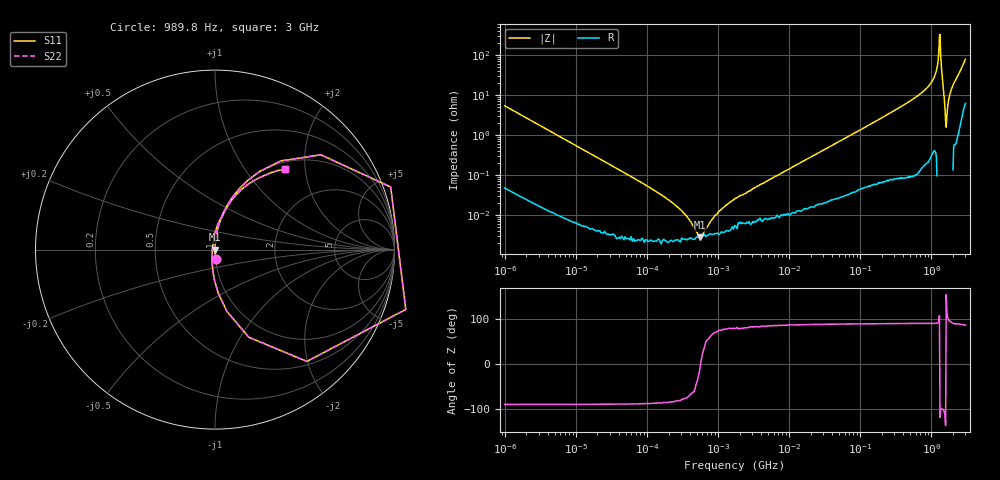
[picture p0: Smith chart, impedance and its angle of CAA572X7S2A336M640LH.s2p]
! S-Parameter Data Generated by TDK Corporation
! Copyright(C) 2020 TDK Corporation.
! All Rights Reserved.
! TDK P/N: CAA572X7S2A336M640LH (Multilayer Ceramic Chip Capacitor)
! Property: C=33uF
! Size(LxWxT): 6x5x6.4mm
! Model Type: s2p (Touchstone File Format Version 1.0)
! Frequency: DC=Yes Start=0.000989846MHz Stop=3000MHz 463points Log-sweep
! Model Generated on Nov. 18, 2020
! Port Assignments:
!  1 ---| |--- 2
! Applicable Conditions:
!  Temperature = 25 degC
!  DC Bias Voltage = 0 V
!  Small Signal Operation
! Terms and conditions regarding TDK Simulation Models
! (1)This simulation model is being provided solely for informational purposes. Please refer to the specifications of the products in terms of detailed characteristics of such products.
! (2)In no event shall TDK Corporation of any of its subsidiaries be liable for any loss or damage arising, directly or indirectly,
!  From any information contained in this simulation model, including, but not limited to loss or damages arising from any inaccuracies, omissions or errors in connection with such information.
! (3)Any and all copyrights on this simulation model are owned by TDK Corporation.
!  Duplication or redistribution of this simulation model without prior written permission from TDK Corporation is prohibited.
! (4)This simulation model is subject to any modification or change without any prior notice.
! (5)Neither TDK Corporation nor any of its subsidiaries shall make any warranty, express or implied,
!  Including but not limited to the correctness, implied warranties of merchantability and fitness for a particular purpose with respect to this simulation models.
! (6)The use of this simulation model shall be deemed to have consented to the terms and conditions hereof.
# Hz S MA R 50
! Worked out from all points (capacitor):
!   462 points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, 989.8 Hz to 3 GHz, reference 50 ohm
!   read as one part in series: C = 29.8 uF near 1.07 kHz
!   lowest |Z| = 2.71 mohm at 550.5 kHz (marker M1)
!   series resonance near 565.4 kHz, so ESL is about 2.7 nH
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989.846  0.05384 -86.4  0.9981 3.1  0.9981 3.1  0.05384 -86.4
12024.64  0.004503 -89.1  0.9999 0.3  0.9999 0.3  0.004503 -89.1
146075.1  0.0003476 -85.9  1 0.0  1 0.0  0.0003476 -85.9
344647  0.0001024 -76.1  1 0.0  1 0.0  0.0001024 -76.1
550451.5  2.709e-05 -13.0  1 0.0  1 0.0  2.709e-05 -13.0
914132.1  9.864e-05 69.6  1 -0.0  1 -0.0  9.864e-05 69.6
1774518  0.0002612 78.5  0.9999 -0.0  0.9999 -0.0  0.0002612 78.5
2.073191e7  0.002892 86.7  0.9998 -0.2  0.9998 -0.2  0.002892 86.7
2.507343e8  0.03376 86.8  0.9987 -1.9  0.9987 -1.9  0.03376 86.8
6.821091e8  0.1035 83.4  0.9934 -5.9  0.9934 -5.9  0.1035 83.4
1.059487e9  0.2406 75.2  0.9671 -13.9  0.9671 -13.9  0.2406 75.2
1.171007e9  0.3735 67.7  0.925 -21.9  0.925 -21.9  0.3735 67.7
1.243477e9  0.6153 53.4  0.8029 -38.0  0.8029 -38.0  0.6153 53.4
1.294266e9  1.039 19.6  0.3495 -86.5  0.3495 -86.5  1.039 19.6
1.374365e9  0.5234 -68.9  0.9473 31.0  0.9473 31.0  0.5234 -68.9
1.430499e9  0.2423 -85.8  1.012 13.8  1.012 13.8  0.2423 -85.8
1.54974e9  0.04582 -111.0  1.017 2.4  1.017 2.4  0.04582 -111.0
1.613037e9  0.01586 152.6  1.014 -0.4  1.014 -0.4  0.01586 152.6
1.782824e9  0.09216 89.7  1.004 -5.3  1.004 -5.3  0.09216 89.7
1.931433e9  0.1474 82.9  0.9926 -8.5  0.9926 -8.5  0.1474 82.9
2.455801e9  0.332 68.5  0.931 -19.4  0.931 -19.4  0.332 68.5
3e9  0.5977 48.9  0.7564 -36.6  0.7564 -36.6  0.5977 48.9
